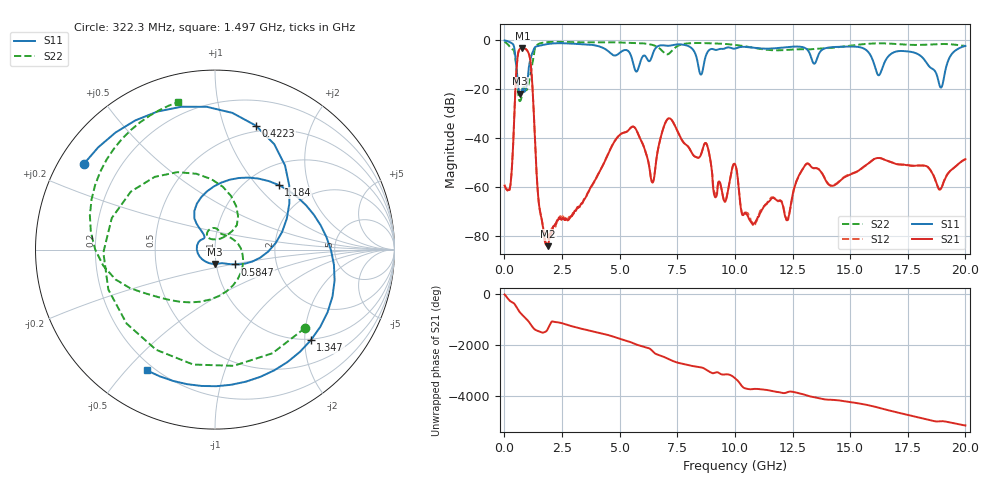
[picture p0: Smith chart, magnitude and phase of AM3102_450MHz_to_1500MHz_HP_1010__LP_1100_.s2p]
!Agilent Technologies,E8364B,MY43040894,A.07.50.67
!Agilent E8364B: A.07.50.67
!Date: Thursday, January 11, 2018 06:20:16
!Correction: S11(Full 2 Port(1,2))
!S21(Full 2 Port(1,2))
!S12(Full 2 Port(1,2))
!S22(Full 2 Port(1,2))
!S2P File: Measurements: S11, S21, S12, S22:
# Hz S  dB  R 50
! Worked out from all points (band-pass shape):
!   1601 points, 10 MHz to 20 GHz, reference 50 ohm
!   highest |S21| = -3.17 dB at 784.6 MHz (marker M1); lowest = -84.3 dB at 1.897 GHz (marker M2)
!   |S21| within 3 dB of the highest: 582.8 MHz to 1.083 GHz (500.5 MHz wide, 60.1 % of centre)
!   lowest |S11| = -21.9 dB at 684.7 MHz (marker M3), VSWR 1.17, Z = 49.2 - j7.96 ohm
!   |S11| at or under -10 dB: 516.4 MHz to 1.079 GHz (562.5 MHz wide, 70.5 % of centre); 16.05 GHz to 16.45 GHz (400.6 MHz wide, 2.47 % of centre); 18.37 GHz to 19.19 GHz (819.6 MHz wide, 4.36 % of centre)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
!   |S22| runs from -24.9 to -0.6 dB; largest |S21 - S12| = 0.00079
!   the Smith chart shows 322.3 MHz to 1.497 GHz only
!   S11 on the Smith chart (normalised r, x): 322.3 MHz: 0.07, +0.29; 422.3 MHz: 0.44, +1.29; 584.7 MHz: 1.23, -0.21; 1.184 GHz: 1.36, +1.32; 1.347 GHz: 0.97, -2.14; 1.497 GHz: 0.17, -0.57
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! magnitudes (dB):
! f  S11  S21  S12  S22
! 10 MHz  -0.1  -59.5  -59.2  -0.6
! 322.3 MHz  -1.2  -52.8  -52.9  -3.5
! 422.3 MHz  -2.8  -33.1  -32.8  -4.4
! 584.7 MHz  -17.2  -6.0  -6.0  -20.2
! 684.7 MHz  -21.9  -3.4  -3.4  -24.9
! 784.6 MHz  -19.9  -3.2  -3.2  -19.5
! 1.184 GHz  -5.9  -14.2  -14.2  -11.1
! 1.347 GHz  -2.7  -44.9  -45.0  -2.8
! 1.497 GHz  -2.2  -66.8  -66.9  -1.4
! 1.897 GHz  -1.5  -84.3  -80.7  -0.7
! 3.346 GHz  -1.6  -67.0  -66.7  -0.8
! 5.045 GHz  -4.8  -38.4  -38.4  -0.9
! 6.419 GHz  -6.1  -58.3  -58.1  -1.9
! 6.682 GHz  -2.3  -43.9  -43.9  -3.0
! 8.743 GHz  -6.3  -42.1  -42.1  -1.2
! 9.555 GHz  -3.4  -66.1  -65.7  -1.5
! 10.01 GHz  -3.4  -50.8  -50.8  -1.9
! 10.8 GHz  -3.1  -75.2  -75.5  -3.0
! 13.34 GHz  -8.0  -52.1  -52.0  -3.6
! 16.68 GHz  -6.4  -49.5  -49.6  -1.3
! 18.94 GHz  -19.4  -60.8  -60.7  -1.5
! 20 GHz  -2.3  -48.7  -48.8  -2.3
